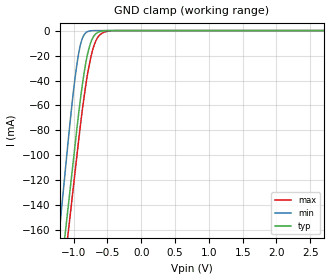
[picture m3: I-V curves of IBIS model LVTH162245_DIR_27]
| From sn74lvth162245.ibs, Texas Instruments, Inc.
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[Model]   LVTH162245_DIR_27
Model_type  Input
Vinl = 0.8
Vinh = 2.0
| variable   typ   min   max
C_comp   3.57pF   2.74pF   4.59pF
[Temperature Range]   40   -40   100
| Ambient temperature   25   -40   85
[Voltage range]   2.7   2.7   2.7
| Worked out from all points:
|   GND clamp passes 1 mA (typ) near -0.62 V on its own axis
[GND Clamp]
| LVTH162245_DIR_27
|   Voltage   I(typ)   I(min)   I(max)
-5.5V     -2.288A    -2.547A    -2.284A
-1.225V   -210.8mA   -168.1mA   -231.1mA
-1.195V   -196.3mA   -151.5mA   -216.7mA
-1.135V   -167.2mA   -118.2mA   -187.9mA
-1.105V   -152.7mA   -101.6mA   -173.6mA
-1.075V   -138.1mA   -84.99mA   -159.2mA
-975mV    -89.73mA   -35.97mA   -111.2mA
-900mV    -54.95mA   -11.36mA   -75.86mA
-775mV    -14.49mA   -458.2uA   -29.04mA
-700mV    -4.229mA   -21.87uA   -12.08mA
-600mV    -595.8uA   -186.1nA   -2.835mA
2.7V      9.09pA     2.798pA    676.8pA
